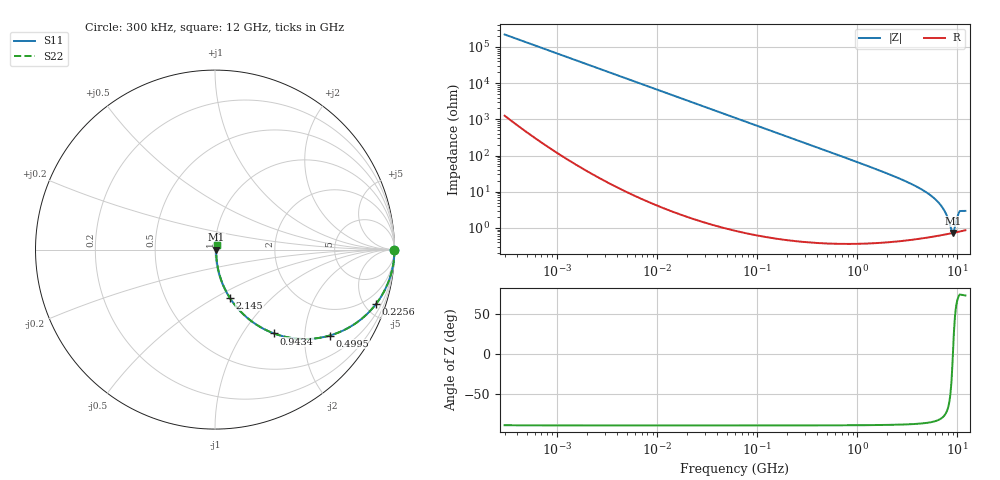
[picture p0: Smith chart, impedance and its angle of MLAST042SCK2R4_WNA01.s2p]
! MLAST042SCK2R4_WNA01  S-PARAMETER MODEL  ( General Type )
! Model Generated by TAIYO YUDEN Corporation (http://www.ty-top.com)
! Version 1.0
! TAIYO YUDEN Control No. 150820
! Copyright(c) 2015 TAIYO YUDEN CO.,LTD. All Rights Reserved.
! Product Description (link to TY-COMPAS)
! https://ds.yuden.co.jp/TYCOMPAS/or/detail?pn=MLAST042SCK2R4AWNA01&u=M
! Products Name : Multilayer Ceramic Capacitors
! Characteristics :
!  Capacitance : 2.4 pF , Rated Voltage : 25V , TCC : CK / C0K
!  Case Size : 0.4 x 0.2 / 0.016 x 0.008 [mm/inch] , Thickness : 0.2 / 0.008 [mm/inch]
!  (Conditions: Temperature = 25 degC , DC Bias Current/Voltage = 0A / 0V)
! External Node Assignments :
!  1  o---| |---o  2
! GND o---------o GND
! Frequency Range : 0.3MHz  -  12000MHz  [ 401 STEP ]
# MHz S RI R 50
! Freq[MHz].  S11 Real  S11 Imag  S21 Real  S21 Imag  S12 Real  S12 Imag  S22 Real  S22 Imag
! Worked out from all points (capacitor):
!   401 points, 300 kHz to 12 GHz, reference 50 ohm
!   read as one part in series: C = 2.39 pF near 316.3 kHz
!   lowest |Z| = 726 mohm at 8.967 GHz (marker M1)
!   series resonance near 9.007 GHz, so ESL is about 130 pH
!   S11 on the Smith chart (normalised r, x): 300 kHz: open; 225.6 MHz: 1.01, -5.90; 499.5 MHz: 1.01, -2.66; 943.4 MHz: 1.01, -1.40; 2.145 GHz: 1.01, -0.59; 12 GHz: 1.02, +0.06
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0.3  1 -0.00045  2.77e-06 0.00045  2.77e-06 0.00045  1 -0.00045
1.769972  1 -0.00266  1.02e-05 0.00266  1.02e-05 0.00266  1 -0.00266
10.44266  0.9997 -0.0157  0.000255 0.0157  0.000255 0.0157  0.9997 -0.0157
60  0.9919 -0.0893  0.00811 0.0893  0.00811 0.0893  0.9919 -0.0893
225.6362  0.8966 -0.3037  0.1034 0.3037  0.1034 0.3037  0.8966 -0.3037
353.9943  0.7789 -0.414  0.2211 0.414  0.2211 0.414  0.7789 -0.414
499.5319  0.6384 -0.4791  0.3616 0.4791  0.3616 0.4791  0.6384 -0.4791
943.3804  0.3288 -0.4672  0.6712 0.4672  0.6712 0.4672  0.3288 -0.4672
1403.667  0.1786 -0.379  0.8214 0.379  0.8214 0.379  0.1786 -0.379
2088.533  0.0866 -0.2746  0.9134 0.2746  0.9134 0.2746  0.0866 -0.2746
2144.601  0.0822 -0.2679  0.9178 0.2679  0.9178 0.2679  0.0822 -0.2679
3944.255  0.0229 -0.1328  0.9771 0.1328  0.9771 0.1328  0.0229 -0.1328
5868.704  0.00995 -0.0644  0.99 0.0644  0.99 0.0644  0.00995 -0.0644
7254.098  0.00743 -0.0319  0.9926 0.0319  0.9926 0.0319  0.00743 -0.0319
7854.144  0.00708 -0.0201  0.9929 0.0201  0.9929 0.0201  0.00708 -0.0201
8503.825  0.00704 -0.00848  0.993 0.00848  0.993 0.00848  0.00704 -0.00848
8966.534  0.00718 -0.000698  0.9928 0.000698  0.9928 0.000698  0.00718 -0.000698
9454.42  0.00746 0.00813  0.9925 -0.00813  0.9925 -0.00813  0.00746 0.00813
9968.853  0.00795 0.018  0.992 -0.018  0.992 -0.018  0.00795 0.018
10511.28  0.00864 0.0276  0.9914 -0.0276  0.9914 -0.0276  0.00864 0.0276
11083.22  0.00891 0.0278  0.9911 -0.0278  0.9911 -0.0278  0.00891 0.0278
12000  0.00932 0.0278  0.9907 -0.0278  0.9907 -0.0278  0.00932 0.0278
